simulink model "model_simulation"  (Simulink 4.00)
settings: Solver=VariableStepDiscrete  StartTime=0.0  StopTime=ts  RelTol=1e-3
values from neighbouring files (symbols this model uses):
  A = [0.9944 -0.1203 -0.4302    [model.m]
  Ao1 = A - K1*c1    [model.m]
  Ao2 = A - K2*c2    [model.m]
  Ao3 = A - K3*c3    [model.m]
  B = [0.4252 -0.0082 0.1813]'    [model.m]
  Bo1 = [B K1]    [model.m]
  Bo2 = [B K2]    [model.m]
  Bo3 = [B K3]    [model.m]
  C = eye(3)    [model.m]
  Co1 = c1    [model.m]
  Co2 = c2    [model.m]
  Co3 = c3    [model.m]
  D = zeros(3,1)    [model.m]
  Do1 = zeros(1,2)    [model.m]
  Do2 = zeros(1,2)    [model.m]
  Do3 = zeros(1,2)    [model.m]
  Tc = 0.1    [model.m]
  tf1 = ts/2    (= 25)    [model.m]
  tf2 = ts/2    (= 25)    [model.m]
  tf3 = ts/2    (= 25)    [model.m]
  x0 = [0.05 0.15 0.2]    [model.m]
libraries: simulink3 x3

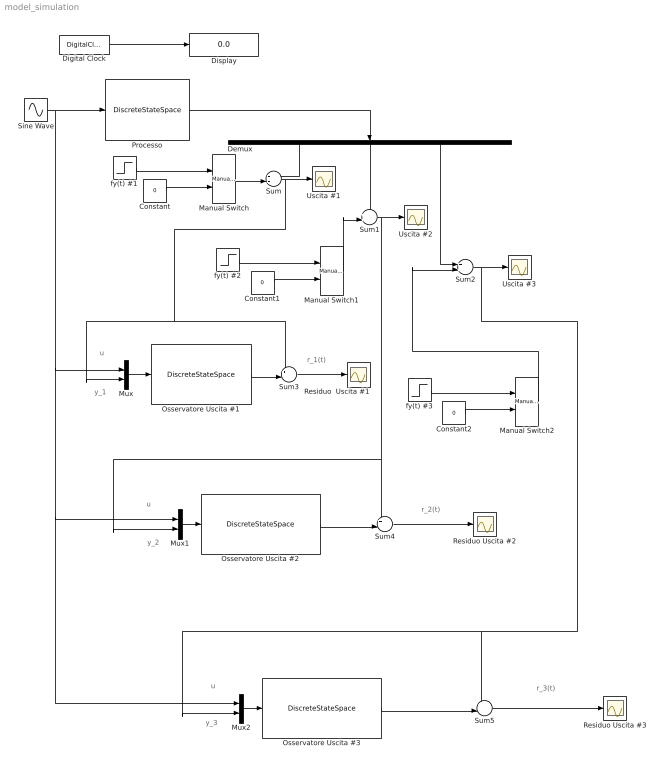
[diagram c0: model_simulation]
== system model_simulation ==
  note: u
  note: y_1
  note: u
  note: y_2
  note: u
  note: y_3
  note: r_1(t)
  note: r_2(t)
  note: r_3(t)
  Constant : Constant  Value=0
  Constant1 : Constant  Value=0
  Constant2 : Constant  Value=0
  Demux : Demux  Orientation=down  Outputs=3  BusSelectionMode=off
  Digital Clock : DigitalClock  SampleTime=0.1
  Display : Display
  Manual Switch : simulink3/Nonlinear/Manual Switch  sw=1  action=0
  Manual Switch1 : simulink3/Nonlinear/Manual Switch  sw=1  action=0
  Manual Switch2 : simulink3/Nonlinear/Manual Switch  sw=1  action=0
  Mux : Mux  Inputs=2
  Mux1 : Mux  Inputs=2
  Mux2 : Mux  Inputs=2
  Osservatore Uscita #1 : DiscreteStateSpace  A=Ao1  B=Bo1  C=Co1  D=Do1  X0=0  SampleTime=Tc  Realization=auto
  Osservatore Uscita #2 : DiscreteStateSpace  A=Ao2  B=Bo2  C=Co2  D=Do2  X0=0  SampleTime=Tc  Realization=auto
  Osservatore Uscita #3 : DiscreteStateSpace  A=Ao3  B=Bo3  C=Co3  D=Do3  X0=0  SampleTime=Tc  Realization=auto
  Processo : DiscreteStateSpace  A=A  B=B  C=C  D=D  X0=x0  SampleTime=Tc  Realization=auto
  Residuo Uscita #2 : Scope
  Residuo Uscita #3 : Scope
  Residuo  Uscita #1 : Scope
  Sine Wave : Sin  SineType=Time-based  Amplitude=1  Bias=0  Frequency=1  Phase=0  Samples=10  SampleTime=Tc
  Sum : Sum  Inputs=++|  SaturateOnIntegerOverflow=on
  Sum1 : Sum  Inputs=++|  SaturateOnIntegerOverflow=on
  Sum2 : Sum  Inputs=++|  SaturateOnIntegerOverflow=on
  Sum3 : Sum  Inputs=+-|  SaturateOnIntegerOverflow=on
  Sum4 : Sum  Inputs=+-|  SaturateOnIntegerOverflow=on
  Sum5 : Sum  Inputs=+-|  SaturateOnIntegerOverflow=on
  Uscita #1 : Scope
  Uscita #2 : Scope
  Uscita #3 : Scope
  fy(t) #1 : Step  Time=tf1  Before=0  After=1  SampleTime=Tc
  fy(t) #2 : Step  Time=tf2  Before=0  After=1  SampleTime=Tc
  fy(t) #3 : Step  Time=tf3  Before=0  After=1  SampleTime=Tc
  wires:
  Sine Wave/1 -> Processo/1, Mux/1, Mux1/1, Mux2/1
  Processo/1 -> Demux/1
  Osservatore Uscita #1/1 -> Sum3/2
  Mux/1 -> Osservatore Uscita #1/1
  Demux/1 -> Sum/1
  Demux/2 -> Sum1/1
  Demux/3 -> Sum2/1
  Digital Clock/1 -> Display/1
  Sum/1 -> Uscita #1/1, Mux/2, Sum3/1
  Sum1/1 -> Uscita #2/1, Mux1/2, Sum4/1
  Sum2/1 -> Uscita #3/1, Mux2/2, Sum5/1
  Sum3/1 -> Residuo  Uscita #1/1
  Osservatore Uscita #2/1 -> Sum4/2
  Mux1/1 -> Osservatore Uscita #2/1
  Sum4/1 -> Residuo Uscita #2/1
  Osservatore Uscita #3/1 -> Sum5/2
  Mux2/1 -> Osservatore Uscita #3/1
  Sum5/1 -> Residuo Uscita #3/1
  fy(t) #1/1 -> Manual Switch/1
  Manual Switch/1 -> Sum/2
  Constant/1 -> Manual Switch/2
  fy(t) #2/1 -> Manual Switch1/1
  Constant1/1 -> Manual Switch1/2
  Manual Switch1/1 -> Sum1/2
  fy(t) #3/1 -> Manual Switch2/1
  Constant2/1 -> Manual Switch2/2
  Manual Switch2/1 -> Sum2/2
